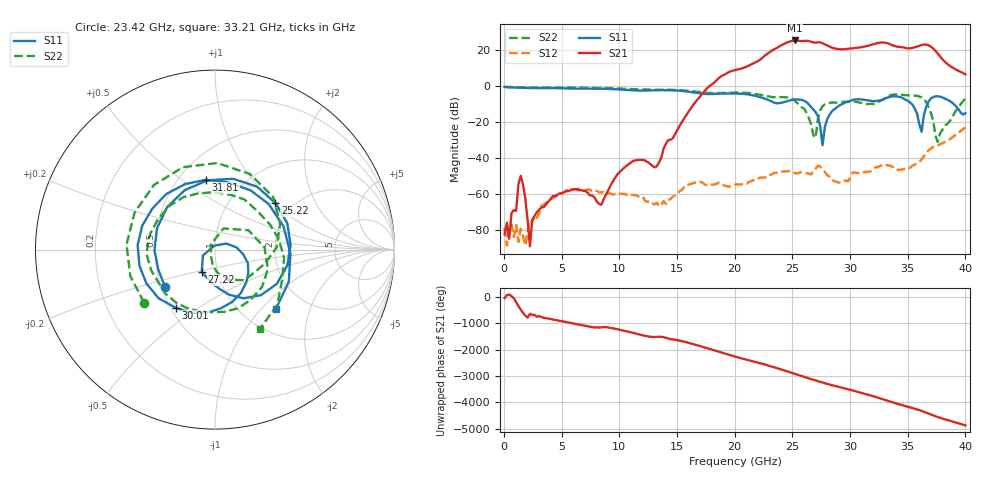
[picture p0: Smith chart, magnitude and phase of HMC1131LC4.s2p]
! Analog Devices, Inc.
! Device:	HMC1131LC4
! Description:	GaAs, pHEMT, MMIC, Medium Power Amplifier, 24 GHz to 35 GHz
! Conditions:	Vdd1 = Vdd2 = Vdd3 = Vdd4 = 5 V
!		Vgg1 = Vgg2 = -1.064 V
!		Idd = 226.6 mA quiescent
!		Pin = -10 dBm
!		Temp = +25 C (EVB baseplate temperature)
! Product validation unit (SN 3) measured on EVB.
! All measurements referenced to the coaxial connectors, except S21a(dB) ref to RFIN pin (i.e., board loss de-embedded from S21a(dB)).
! Freq(GHz)	S11a(dB)	S11p(deg)	S21a(dB)	S21p(deg)	S12a(dB)	S12p(deg)	S22a(dB)	S22p(deg)
# GHz S DB R 50
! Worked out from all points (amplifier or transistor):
!   201 points, 50 MHz to 40 GHz, reference 50 ohm
!   highest |S21| = 25.4 dB at 25.22 GHz (marker M1)
!   |S21| within 3 dB of that: 23.96 GHz to 28.09 GHz (4.129 GHz wide, 15.9 % of centre)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
!   unconditionally stable (mu >= 1): start of sweep to end of sweep
!   at 6.642 GHz: K = 13146.42, MAG = -44.5 dB, |S12| = -57.2 dB
!   at 20.02 GHz: K = 33.71, MAG = 13.6 dB, |S12| = -54.8 dB
!   at 40 GHz: K = 2.67, MAG = 7.7 dB, |S12| = -23.0 dB
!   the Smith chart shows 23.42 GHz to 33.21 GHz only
!   S11 on the Smith chart (normalised r, x): 23.42 GHz: 0.52, -0.25; 25.22 GHz: 1.61, +1.02; 27.22 GHz: 0.84, -0.21; 30.01 GHz: 0.53, -0.41; 31.81 GHz: 0.68, +0.62; 33.21 GHz: 1.41, -1.21
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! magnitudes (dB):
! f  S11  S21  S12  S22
! 50 MHz  -0.4  -82.4  -79.0  -0.4
! 1.049 GHz  -0.7  -69.4  -77.3  -0.5
! 1.448 GHz  -0.9  -49.9  -79.4  -0.6
! 2.247 GHz  -1.0  -89.0  -74.6  -0.7
! 6.841 GHz  -1.4  -58.2  -57.7  -0.8
! 8.44 GHz  -1.4  -65.9  -59.1  -1.0
! 10.84 GHz  -2.2  -43.2  -60.1  -1.5
! 13.43 GHz  -2.2  -42.5  -66.7  -1.9
! 20.02 GHz  -4.1  8.9  -54.8  -3.6
! 23.42 GHz  -9.2  20.6  -48.2  -6.1
! 25.22 GHz  -7.4  25.4  -48.4  -8.2
! 26.82 GHz  -12.9  24.4  -47.4  -27.3
! 27.22 GHz  -16.8  24.5  -44.3  -17.9
! 27.62 GHz  -32.9  23.9  -46.5  -11.2
! 28.21 GHz  -16.0  22.0  -50.3  -9.3
! 30.01 GHz  -8.2  20.9  -50.9  -8.5
! 31.81 GHz  -8.1  22.9  -47.2  -9.8
! 33.21 GHz  -6.5  24.0  -43.9  -5.9
! 33.41 GHz  -6.0  23.5  -44.2  -5.2
! 36.2 GHz  -25.3  22.9  -40.8  -6.2
! 37.6 GHz  -5.6  18.2  -32.9  -31.0
! 40 GHz  -15.0  6.6  -23.0  -6.7
